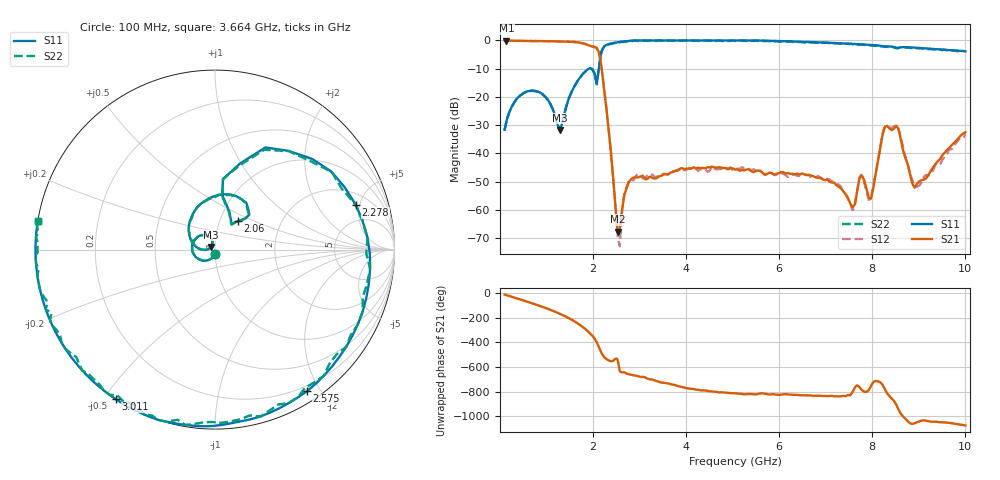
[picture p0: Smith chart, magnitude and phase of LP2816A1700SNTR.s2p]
!	AVX	THIN	FILM	OPERATION
!	LP2816S	High	Performance	Low	Pass	Filters
!	P/N	LP2816A1700SNTR
!	Created	10	January	2017
!Instrument:	"HEWLETT PACKARD,8720ES,US39172150,7.62 "
#	MHz	S	dB	R	50
!	Frq	S11(dB)	S11(deg)	S21(dB)	S21(deg)	S12(dB)	S12(deg)	S22(dB)	S22(deg)
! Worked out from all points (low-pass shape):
!   501 points, 100 MHz to 10 GHz, reference 50 ohm
!   highest |S21| = -0.05 dB at 139.6 MHz (marker M1); lowest = -67.7 dB at 2.535 GHz (marker M2)
!   |S21| within 3 dB of the highest: start of sweep to 2.091 GHz
!   lowest |S11| = -31.7 dB at 1.288 GHz (marker M3), VSWR 1.05, Z = 47.9 + j1.39 ohm
!   |S11| at or under -10 dB: start of sweep to 1.912 GHz; 1.966 GHz to 2.123 GHz (157 MHz wide, 7.68 % of centre)
!   |S22| runs from -31.9 to 0.0 dB; largest |S21 - S12| = 0.021
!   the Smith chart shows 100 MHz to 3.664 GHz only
!   S11 on the Smith chart (normalised r, x): 100 MHz: 1.00, -0.05; 2.06 GHz: 1.22, +0.40; 2.278 GHz: 2.98, +4.60; 2.575 GHz: 0.13, -1.84; 3.011 GHz: -0.00, -0.54; 3.664 GHz: -0.00, +0.08
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100  -31.68 -93.3  -0.05 -11.7  -0.03 -11.7  -31.78 -93.5
139.6  -28.68 -100.8  -0.05 -16.3  -0.04 -16.4  -28.78 -100.9
753.4  -17.83 159.8  -0.23 -90.6  -0.20 -90.4  -18.03 159.7
1288  -31.73 145.8  -0.35 -168.2  -0.32 -168.3  -31.93 145.6
1525.6  -18.71 168.5  -0.46 147.2  -0.44 146.8  -18.81 168.4
1763.2  -12.21 117.1  -0.95 88.9  -1.01 89.3  -12.21 117.1
2060.2  -13.85 51.3  -2.52 -26.7  -2.50 -27.6  -13.95 51.2
2159.2  -6.01 73.7  -7.16 -107.3  -7.42 -109.0  -6.21 73.7
2278  -1.69 17.6  -22.81 -173.2  -22.43 -171.9  -1.69 17.6
2535.4  -0.65 -49.0  -67.71 166.0  -70.23 173.5  -0.65 -49.2
2575  -0.53 -56.9  -66.51 84.7  -72.90 106.2  -0.73 -57.0
2713.6  -0.29 -81.3  -52.64 67.2  -52.34 70.6  -0.39 -81.5
3010.6  0.00 -123.6  -48.25 38.5  -47.83 34.3  -0.20 -123.8
3406.6  0.00 -166.4  -48.28 0.2  -47.73 1.6  0.00 -166.5
3664  0.00 170.8  -46.81 -20.2  -46.46 -22.6  0.00 170.7
5050  0.00 83.8  -45.76 -94.2  -45.54 -85.8  -0.20 83.7
6713.2  -0.60 7.4  -48.01 -114.3  -48.54 -111.9  -0.80 7.3
7762.6  -1.42 -38.3  -48.05 -62.5  -47.56 -66.4  -1.42 -38.3
7940.8  -1.57 -46.4  -55.84 -56.7  -56.24 -58.7  -1.67 -46.4
8356.6  -2.10 -63.9  -31.03 -113.2  -30.60 -119.9  -2.20 -64.1
8950.6  -2.60 -89.4  -51.05 29.0  -51.88 29.6  -2.80 -89.5
10000  -3.84 -143.6  -32.55 4.0  -33.21 9.3  -3.84 -143.8
